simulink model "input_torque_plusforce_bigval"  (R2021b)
settings: Solver=VariableStepAuto  StartTime=0.0  StopTime=2  RelTol=1e-3
undefined symbols (not defined in the file or in its folder): BLDC, dynamics
libraries: fl_lib x20, nesl_utility x7, sdl_lib x1

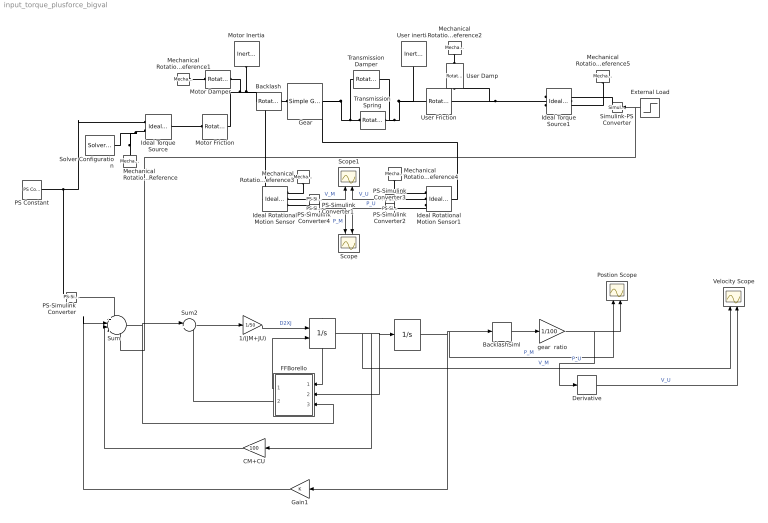
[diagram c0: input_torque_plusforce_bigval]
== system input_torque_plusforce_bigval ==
  " " : Integrator  ExternalReset=rising  ShowStatePort=on
  "  " : Integrator  UpperSaturationLimit=dynamics.ThUmax/dynamics.tau  LowerSaturationLimit=dynamics.ThUmin/dynamics.tau
  " Gear" : sdl_lib/Gears/Simple Gear  ratio=100  rotation_direction=sdl.enum.shaftOutputDirection.same  friction_model=sdl.enum.gear_efficiencies_load.off  T_noload=0.1 N*m  T_nom=5 N*m  efficiency_nom=0.8  efficiency=0.8  temperature_TLU=[280, 300, 320] K  load_TLU=[1, 5, 10] N*m  efficiency_TLU=[.95, .9, .85]  efficiency_TLU2=[.85, .8, .75; .95, .9, .85; .85, .8, .7]  w_thr=0.01 rad/s  pwr_thr=0.001 W  backlash_model=sdl.enum.backlashModel.Off  backlash_distance=1e-3 mm  x0=0 mm  r_base=0.1 m  hardstop_model=simscape.enum.hardstop.smooth  transition=1e-4 mm  backlash_stiffness=1e7 N/m  backlash_damping=1e6 N/(m/s)  e=0  v_tol=0.001 m/s  mu_visc=[0, 0] N*m/(rad/s)  enable_faults=simscape.enum.onoff.off  efficiency_fault=0.05  external_fault=simscape.enum.onoff.off  temporal_fault=simscape.enum.onoff.off  fault_time=5 s  fault_angles=pi / 12 rad  report_fault=simscape.enum.assert.action.none  thermal_mass=50 J/K  temperature_specify=off  temperature_priority=High  temperature=300 K  temperature_nominal_specify=off  temperature_nominal_unit=K  temperature_nominal_value=1
  1/(JM+JU) : Gain  Gain=1/50
  Backlash : fl_lib/Mechanical/Rotational Elements/Rotational Hard Stop  upper_bnd=1%1e-10%1 deg  lower_bnd=-1%1e-11%-1 deg  stiff_up=1e6 N*m/rad  stiff_low=1e6 N*m/rad  D_up=0.01 N*m/(rad/s)  D_low=0.01 N*m/(rad/s)  model=simscape.enum.hardstop.smooth  transition=0.001 rad  w_specify=off  w_priority=None  w=0 rad/s  w_nominal_specify=off  w_nominal_unit=rad/s  w_nominal_value=1  t_specify=off  t_priority=None  t=0 N*m  t_nominal_specify=off  t_nominal_unit=N*m  t_nominal_value=1  phi_specify=off  phi_priority=High  phi=0 rad  phi_nominal_specify=off  phi_nominal_unit=rad  phi_nominal_value=1
  BacklashSiml : Backlash  BacklashWidth=1/57
  CM+CU : Gain  Gain=100
  Derivative : Derivative
  External Load : Step  Time=1.4  After=100  SampleTime=0
  FFBorello : Subsystem
  Gain1 : Gain
  Ideal Rotational Motion Sensor : fl_lib/Mechanical/Mechanical Sensors/Ideal Rotational Motion Sensor  wrap_angle=simscape.enum.onoff.off  offset=0 rad
  Ideal Rotational Motion Sensor1 : fl_lib/Mechanical/Mechanical Sensors/Ideal Rotational Motion Sensor  wrap_angle=simscape.enum.onoff.off  offset=0 rad
  Ideal Torque Source : fl_lib/Mechanical/Mechanical Sources/Ideal Torque Source
  Ideal Torque Source1 : fl_lib/Mechanical/Mechanical Sources/Ideal Torque Source
  Mechanical Rotational Reference{,1..5} (6 alike) : fl_lib/Mechanical/Rotational Elements/Mechanical Rotational Reference
  Motor Damper : fl_lib/Mechanical/Rotational Elements/Rotational Damper  D=0.03 N*m/(rad/s)  w_specify=off  w_priority=None  w=0 rad/s  w_nominal_specify=off  w_nominal_unit=rad/s  w_nominal_value=1  t_specify=off  t_priority=None  t=0 N*m  t_nominal_specify=off  t_nominal_unit=N*m  t_nominal_value=1
  Motor Friction : fl_lib/Mechanical/Rotational Elements/Rotational Friction  brkwy_trq=5 N*m  brkwy_vel=0.1 rad/s  Col_trq=5 N*m  visc_coef=0 N*m/(rad/s)  w_specify=off  w_priority=None  w=0 rad/s  w_nominal_specify=off  w_nominal_unit=rad/s  w_nominal_value=1  t_specify=off  t_priority=None  t=0 N*m  t_nominal_specify=off  t_nominal_unit=N*m  t_nominal_value=1
  Motor Inertia : fl_lib/Mechanical/Rotational Elements/Inertia  inertia=0.085 kg*m^2  num_ports=foundation.enum.numPorts2.one  w_specify=off  w_priority=High  w=0 rad/s  w_nominal_specify=off  w_nominal_unit=rad/s  w_nominal_value=1  t_specify=off  t_priority=None  t=0 N*m  t_nominal_specify=off  t_nominal_unit=N*m  t_nominal_value=1
  PS Constant : fl_lib/Physical Signals/Sources/PS Constant  constant=4 N*m
  PS-Simulink Converter{,1..4} (5 alike) : nesl_utility/PS-Simulink Converter  PhysicalDomain=network_engine_domain  SubClassName=ps_output  LeftPortType=input  RightPortType=output  PseudoPeriodic=off  Frequencies=[]  Unit=inherit  AffineConversion=off
  Postion Scope : Scope  NumInputPorts=2
  Scope : Scope  NumInputPorts=2
  Scope1 : Scope  NumInputPorts=2
  Simulink-PS Converter : nesl_utility/Simulink-PS Converter  PhysicalDomain=network_engine_domain  SubClassName=ps_input  LeftPortType=input  RightPortType=output  PseudoPeriodic=off  Frequencies=[]  NoiseDistribution=none  NoiseParameters=[]  Unit=1  AffineConversion=off  FilteringAndDerivatives=provide  SimscapeFilterOrder=1  InputFilterTimeConstant=0.001  UdotUserProvided=0
  Solver Configuration : nesl_utility/Solver Configuration  PhysicalDomain=network_engine_domain  SubClassName=solver  LeftPortType=input  RightPortType=generic  Tones=[]  Harmonics=[]  SimulateNoise=off  Profile=off  UseLocalSampling=off  EnableSwitchedLinearOptims=on  FrequencyDomain=off  UseCCode=off  RelTol=0.001  AbsTol=1e-06  MinStep=1e-09  ToWorkspace=off  RevertToSquareIcSolve=off  NumHomotopyIterations=100  PhasorMode=off  PhasorModeNumHarmonics=1  DoDC=off  ResidualTolerance=1e-09  UseLocalSolver=off  LocalSolverChoice=NE_BACKWARD_EULER_ADVANCER  LocalSolverSampleTime=0.001  DoFixedCost=off  MaxNonlinIter=3  MaxModeIter=2  ComputeImpulses=off  ImpulseIterations=2  LinearAlgebra=auto  EquationFormulation=NE_TIME_EF  DelaysMemoryBudget=1024  AutomaticFiltering=on  FilteringTimeConstant=0.001  PartitionStorageMethod=AS_NEEDED  PartitionMemoryBudget=1024  PartitionMethod=ROBUST
  Sum : Sum  Inputs=+---
  Sum2 : Sum  Inputs=|+-
  Transmission Damper : fl_lib/Mechanical/Rotational Elements/Rotational Damper  D=500 N*m/(rad/s)  w_specify=off  w_priority=None  w=0 rad/s  w_nominal_specify=off  w_nominal_unit=rad/s  w_nominal_value=1  t_specify=off  t_priority=None  t=0 N*m  t_nominal_specify=off  t_nominal_unit=N*m  t_nominal_value=1
  Transmission Spring : fl_lib/Mechanical/Rotational Elements/Rotational Spring  spr_rate=1e5 N*m/rad  w_specify=off  w_priority=None  w=0 rad/s  w_nominal_specify=off  w_nominal_unit=rad/s  w_nominal_value=1  t_specify=off  t_priority=None  t=0 N*m  t_nominal_specify=off  t_nominal_unit=N*m  t_nominal_value=1  phi_specify=off  phi_priority=High  phi=0 rad  phi_nominal_specify=off  phi_nominal_unit=rad  phi_nominal_value=1
  User Damp : fl_lib/Mechanical/Rotational Elements/Rotational Damper  D=100 N*m/(rad/s)  w_specify=off  w_priority=None  w=0 rad/s  w_nominal_specify=off  w_nominal_unit=rad/s  w_nominal_value=1  t_specify=off  t_priority=None  t=0 N*m  t_nominal_specify=off  t_nominal_unit=N*m  t_nominal_value=1
  User Friction : fl_lib/Mechanical/Rotational Elements/Rotational Friction  brkwy_trq=500 N*m  brkwy_vel=0.1 rad/s  Col_trq=500 N*m  visc_coef=0 N*m/(rad/s)  w_specify=off  w_priority=None  w=0 rad/s  w_nominal_specify=off  w_nominal_unit=rad/s  w_nominal_value=1  t_specify=off  t_priority=None  t=0 N*m  t_nominal_specify=off  t_nominal_unit=N*m  t_nominal_value=1
  User inertia : fl_lib/Mechanical/Rotational Elements/Inertia  inertia=50 kg*m^2  num_ports=foundation.enum.numPorts2.one  w_specify=off  w_priority=High  w=0 rad/s  w_nominal_specify=off  w_nominal_unit=rad/s  w_nominal_value=1  t_specify=off  t_priority=None  t=0 N*m  t_nominal_specify=off  t_nominal_unit=N*m  t_nominal_value=1
  Velocity Scope : Scope  NumInputPorts=2
  gear  ratio : Gain  Gain=1/100
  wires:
  CM+CU/1 -> Sum/3
  External Load/1 -> Sum/4, Simulink-PS Converter/1
  PS-Simulink Converter/1 -> Sum/1
  BacklashSiml/1 -> gear  ratio/1
  gear  ratio/1 -> Postion Scope/2, Derivative/1  "P_U"
  PS-Simulink Converter1/1 -> Scope/1  "P_M"
  PS-Simulink Converter3/1 -> Scope/2  "P_U"
  Gain1/1 -> Sum/2
  1/(JM+JU)/1 -> " "/1  "D2XJ"
  Derivative/1 -> Velocity Scope/2  "V_U"
  " "/1 -> Velocity Scope/1, CM+CU/1, "  "/1, FFBorello/2(DXJ)  "V_M"
  "  "/1 -> Gain1/1, Postion Scope/1, BacklashSiml/1  "P_M"
  " "/State -> FFBorello/1(DXJ SP)
  FFBorello/2(TF) -> Sum2/2
  Sum2/1 -> 1/(JM+JU)/1
  FFBorello/1(Reset_DXJ) -> " "/2
  PS-Simulink Converter4/1 -> Scope1/1  "V_M"
  PS-Simulink Converter2/1 -> Scope1/2  "V_U"
  Sum/1 -> FFBorello/3(Act Torque), Sum2/1
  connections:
  Ideal Torque Source/RConn2 -- Mechanical Rotational Reference/LConn1 -- Solver Configuration/RConn1
  Transmission Spring/RConn1 -- Transmission Damper/RConn1 -- User Friction/LConn1 -- User inertia/LConn1
  Ideal Torque Source1/LConn1 -- User Friction/RConn1 -- User Damp/RConn1
  Motor Inertia/LConn1 -- Motor Friction/RConn1 -- Motor Damper/RConn1 -- Ideal Rotational Motion Sensor/LConn1 -- Backlash/LConn1
  Transmission Spring/LConn1 -- Transmission Damper/LConn1 -- Ideal Rotational Motion Sensor1/LConn1 -- " Gear"/RConn1
  PS-Simulink Converter/LConn1 -- PS Constant/RConn1 -- Ideal Torque Source/RConn1
  Ideal Rotational Motion Sensor1/RConn3 -- PS-Simulink Converter3/LConn1
  Simulink-PS Converter/RConn1 -- Ideal Torque Source1/RConn1
  Backlash/RConn1 -- " Gear"/LConn1
  Mechanical Rotational Reference3/LConn1 -- Ideal Rotational Motion Sensor/RConn1
  PS-Simulink Converter4/LConn1 -- Ideal Rotational Motion Sensor/RConn2
  Mechanical Rotational Reference5/LConn1 -- Ideal Torque Source1/RConn2
  Mechanical Rotational Reference1/LConn1 -- Motor Damper/LConn1
  Mechanical Rotational Reference4/LConn1 -- Ideal Rotational Motion Sensor1/RConn1
  PS-Simulink Converter1/LConn1 -- Ideal Rotational Motion Sensor/RConn3
  Motor Friction/LConn1 -- Ideal Torque Source/LConn1
  PS-Simulink Converter2/LConn1 -- Ideal Rotational Motion Sensor1/RConn2
  Mechanical Rotational Reference2/LConn1 -- User Damp/LConn1

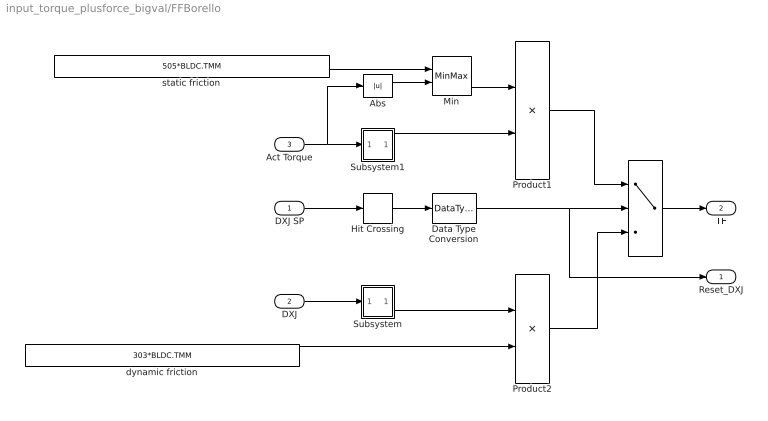
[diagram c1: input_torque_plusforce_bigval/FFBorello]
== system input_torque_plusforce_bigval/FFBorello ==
  DXJ SP : Inport
  DXJ : Inport  Port=2
  Act Torque : Inport  Port=3
  "   " : Switch  Threshold=0.5
  Abs : Abs
  Data Type Conversion : DataTypeConversion  OutDataTypeStr=double
  Hit Crossing : HitCross
  Min : MinMax  Inputs=2  InputSameDT=on  SaturateOnIntegerOverflow=on
  Product1 : Product  InputSameDT=on  RndMeth=Zero  SaturateOnIntegerOverflow=on
  Product2 : Product  InputSameDT=on  RndMeth=Zero  SaturateOnIntegerOverflow=on
  Subsystem : Subsystem
  Subsystem1 : Subsystem
  dynamic friction : Constant  Value=303*BLDC.TMM
  static friction : Constant  Value=505*BLDC.TMM
  Reset_DXJ : Outport
  TF : Outport  Port=2
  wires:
  Product2/1 -> "   "/3
  DXJ/1 -> Subsystem/1(In1)
  "   "/1 -> TF/1
  Product1/1 -> "   "/1
  Min/1 -> Product1/1
  Act Torque/1 -> Subsystem1/1(In1), Abs/1
  Abs/1 -> Min/2
  Hit Crossing/1 -> Data Type Conversion/1
  Subsystem/1(Out1) -> Product2/1
  Subsystem1/1(Out1) -> Product1/2
  Data Type Conversion/1 -> "   "/2, Reset_DXJ/1
  DXJ SP/1 -> Hit Crossing/1
  static friction/1 -> Min/1
  dynamic friction/1 -> Product2/2

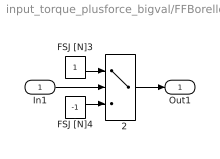
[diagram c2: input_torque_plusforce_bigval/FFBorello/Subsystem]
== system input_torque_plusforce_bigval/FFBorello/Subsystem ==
  In1 : Inport
  "   2" : Switch
  FSJ [N]3 : Constant
  FSJ [N]4 : Constant  Value=-1
  Out1 : Outport
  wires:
  FSJ [N]3/1 -> "   2"/1
  FSJ [N]4/1 -> "   2"/3
  In1/1 -> "   2"/2
  "   2"/1 -> Out1/1

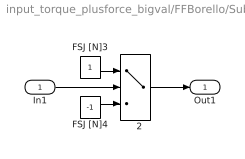
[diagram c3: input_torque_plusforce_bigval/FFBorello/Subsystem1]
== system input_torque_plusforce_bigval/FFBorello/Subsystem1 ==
  In1 : Inport
  "   2" : Switch
  FSJ [N]3 : Constant
  FSJ [N]4 : Constant  Value=-1
  Out1 : Outport
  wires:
  FSJ [N]3/1 -> "   2"/1
  FSJ [N]4/1 -> "   2"/3
  In1/1 -> "   2"/2
  "   2"/1 -> Out1/1
